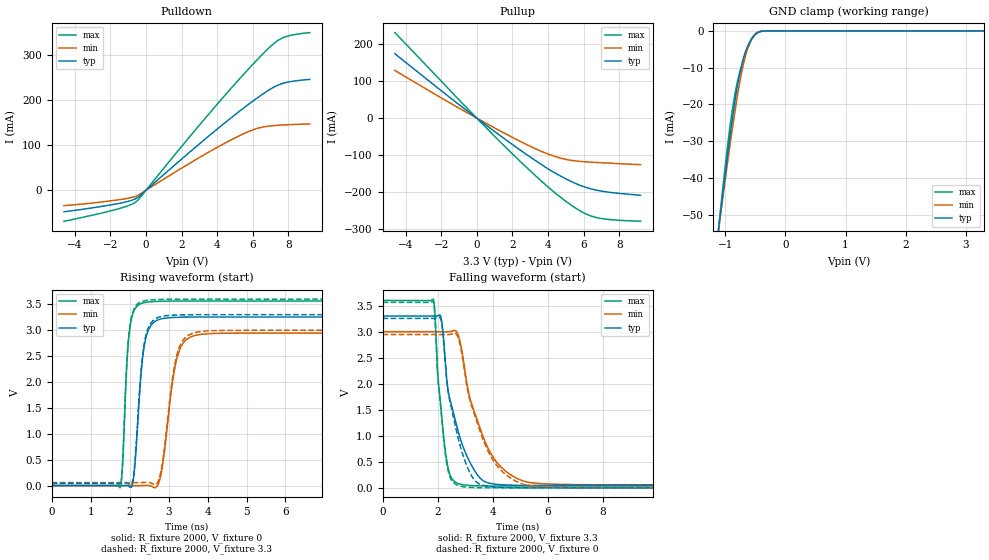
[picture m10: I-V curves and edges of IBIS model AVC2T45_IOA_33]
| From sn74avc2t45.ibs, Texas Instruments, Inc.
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[Model]   AVC2T45_IOA_33
Model_type  I/O
Vinl=0.8
Vinh=2.0
Enable   Active-Low
Vref =   0
Rref =   2000
Cref =   15p
Vmeas =   1.65
| variable   typ   min   max
C_comp   4.80pF   3.94pF   5.78pF
| C_pullup   3.85pF   2.95pF   5.15pF
| C_pulldown   4.06pF   3.58pF   4.64pF
| C_tri-state   4.80pF   3.94pF   5.78pF
[Temperature Range]   40   100   -40
| Ambient temperature   25   85   -40
[Voltage range]   3.3   3   3.6
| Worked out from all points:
|   slope of the pulldown table from 0 to 0.495 V, typ, clamps not added: 28.7 ohm
|   slope of the pullup table from 0 to 0.495 V, typ, clamps not added: 27.4 ohm
|   GND clamp passes 1 mA (typ) near -0.50 V on its own axis
|   rising waveform, R_fixture 2000, V_fixture 0: 20-80 % time 197ps typ, 301ps min, 138ps max; typ from 0 V to 3.26 V
|   falling waveform, R_fixture 2000, V_fixture 3.3: 20-80 % time 746ps typ, 1ns min, 326ps max; typ from 3.3 V to 0.046 V
|   rising waveform, R_fixture 2000, V_fixture 3.3: 20-80 % time 196ps typ, 297ps min, 138ps max; typ from 0.046 V to 3.3 V
|   falling waveform, R_fixture 2000, V_fixture 0: 20-80 % time 659ps typ, 1ns min, 322ps max; typ from 3.26 V to 0 V
[GND Clamp]
| AVC2T45_IOA_33
|   Voltage   I(typ)   I(min)   I(max)
-4.6V     -597.8mA   -546.6mA   -662.5mA
-1.12V    -54.88mA   -55.04mA   -54.73mA
-1.09V    -50.72mA   -51.27mA   -50.03mA
-1V       -38.53mA   -40.19mA   -36.43mA
-920mV    -28.25mA   -30.71mA   -25.57mA
-870mV    -22.29mA   -25.06mA   -19.99mA
-810mV    -15.96mA   -18.69mA   -14.59mA
-725mV    -9.083mA   -10.96mA   -9.257mA
-630mV    -4.179mA   -4.838mA   -4.797mA
-545mV    -1.809mA   -1.649mA   -1.862mA
-450mV    -412.7uA   -343uA     -301.7uA
3.3V      1.631nA    2.406uA    228.2pA
[Pulldown]
| AVC2T45_IOA_33
|   Voltage   I(typ)   I(min)   I(max)
-4.6V     -47.48mA   -33.99mA   -68.59mA
-1.68V    -30.25mA   -21.7mA    -42.42mA
-975mV    -24.15mA   -17.32mA   -33.81mA
-545mV    -17.86mA   -12.84mA   -25.24mA
2.54V     87.35mA    61.85mA    122.6mA
4.5V      151.6mA    105.9mA    213.3mA
5.905V    194.7mA    132.4mA    274.8mA
6.805V    219.6mA    141.6mA    311.5mA
7.315V    231.2mA    143.7mA    329.3mA
7.73V     237.3mA    144.7mA    338.5mA
8.275V    241.7mA    145.7mA    344.4mA
9.2V      245.6mA    146.9mA    349.3mA
[Pullup]
| AVC2T45_IOA_33
|   Voltage   I(typ)   I(min)   I(max)
-4.6V     174.2mA    129.1mA    231.4mA
-1.105V   40.58mA    29.86mA    54.82mA
1.58V     -56.83mA   -41.58mA   -76.89mA
3.53V     -122.6mA   -88.07mA   -166.1mA
4.725V    -157.4mA   -108.5mA   -215.1mA
5.775V    -181.6mA   -117mA     -250.3mA
6.525V    -192.9mA   -119.7mA   -266.7mA
7.46V     -201mA     -122mA     -274.6mA
9.2V      -209mA     -126mA     -279.3mA
[Ramp]
| AVC2T45_IOA_33
| variable   typ   min   max
dV/dt_r   1.98/2.02E-10   1.79/3.12E-10   2.17/1.41E-10
dV/dt_f   1.97/7.47E-10   1.78/1.00E-09   2.15/3.28E-10
R_load = 2000
[Rising Waveform]
| AVC2T45_IOA_33
R_fixture =   2000
C_fixture =   0
L_fixture =   0
V_fixture =   0
V_fixture_min = 0
V_fixture_max = 0
|   Time   V(typ)   V(min)   V(max)
0s        38.02nV    120.5nV    1.934nV
1.755ns   -24.17uV   -4.743uV   -43.6mV
2.015ns   -32.39mV   33.42uV    3.087V
2.11ns    201.9mV    25.71uV    3.369V
2.31ns    2.296V     324.5uV    3.518V
2.46ns    2.962V     4.618mV    3.543V
2.785ns   3.214V     150.3mV    3.559V
3.275ns   3.25V      2.607V     3.563V
3.86ns    3.255V     2.923V     3.564V
34.99ns   3.256V     2.946V     3.564V
[Falling Waveform]
| AVC2T45_IOA_33
R_fixture =   2000
C_fixture =   0
L_fixture =   0
V_fixture =   3.3
V_fixture_min = 3
V_fixture_max = 3.6
|   Time   V(typ)   V(min)   V(max)
0s        3.3V       3V         3.6V
1.845ns   3.299V     3V         3.626V
2.13ns    3.263V     2.999V     1.502V
2.325ns   2.145V     2.996V     549.8mV
2.695ns   1.199V     2.999V     95.88mV
2.895ns   839.4mV    2.599V     63.03mV
3.19ns    480mV      1.698V     45.43mV
3.88ns    90.07mV    715mV      37.25mV
5.365ns   47.39mV    101mV      36.36mV
34.99ns   46.48mV    58.85mV    36.33mV
[Rising Waveform]
| AVC2T45_IOA_33
R_fixture =   2000
C_fixture =   0
L_fixture =   0
V_fixture =   3.3
V_fixture_min = 3
V_fixture_max = 3.6
|   Time   V(typ)   V(min)   V(max)
0s        46.48mV    58.85mV    36.33mV
1.755ns   46.45mV    58.85mV    -7.402mV
2.01ns    15.35mV    58.88mV    3.099V
2.11ns    249.5mV    58.88mV    3.405V
2.31ns    2.349V     59.18mV    3.554V
2.46ns    3.01V      63.48mV    3.579V
2.785ns   3.259V     211.3mV    3.595V
3.265ns   3.294V     2.651V     3.599V
3.85ns    3.299V     2.977V     3.6V
34.99ns   3.3V       3V         3.6V
[Falling Waveform]
| AVC2T45_IOA_33
R_fixture =   2000
C_fixture =   0
L_fixture =   0
V_fixture =   0
V_fixture_min = 0
V_fixture_max = 0
|   Time   V(typ)   V(min)   V(max)
0s        3.256V     2.946V     3.564V
1.845ns   3.254V     2.946V     3.59V
2.13ns    3.219V     2.945V     1.46V
2.32ns    2.139V     2.942V     514.1mV
2.69ns    1.089V     2.948V     59.34mV
2.895ns   677.8mV    2.543V     26.02mV
3.185ns   283.2mV    1.663V     9mV
3.875ns   26.15mV    662.4mV    912.4uV
5.33ns    569.5uV    42.39mV    32.56uV
34.99ns   487.1nV    724.6nV    210.5nV
